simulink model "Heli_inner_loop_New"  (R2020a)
settings: Solver=FixedStepDiscrete  StartTime=0.0  StopTime=10.0  FixedStep=0.01  RelTol=1e-3  EnableMultiTasking=on
libraries: HeliLibrary_New x3, simulink x1

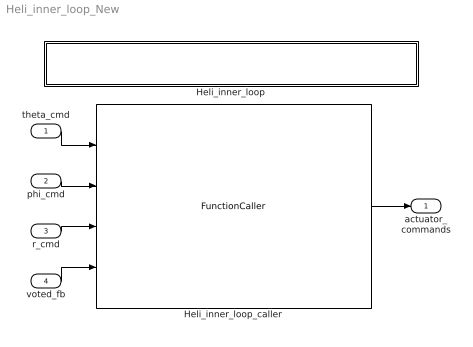
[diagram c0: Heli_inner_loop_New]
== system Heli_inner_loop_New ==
  theta_cmd : Inport  OutMin=-30  OutMax=30  OutDataTypeStr=double  PortDimensions=1  SampleTime=0.01
  phi_cmd : Inport  Port=2  OutMin=-30  OutMax=30  OutDataTypeStr=double  PortDimensions=1  SampleTime=0.01
  r_cmd : Inport  Port=3  OutMin=-30  OutMax=30  OutDataTypeStr=double  PortDimensions=1  SampleTime=0.01
  voted_fb : Inport  Port=4  OutMin=-180  OutMax=180  OutDataTypeStr=double  PortDimensions=5  SampleTime=0.01
  Heli_inner_loop : Subsystem  TreatAsAtomicUnit=on
  Heli_inner_loop_caller : FunctionCaller  FunctionPrototype=actuator_commands = Heli_inner_loop(theta_cmd,phi_cmd,r_cmd,voted_fb)
  actuator_commands : Outport  VectorParamsAs1DForOutWhenUnconnected=off
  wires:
  voted_fb/1 -> Heli_inner_loop_caller/4
  r_cmd/1 -> Heli_inner_loop_caller/3
  phi_cmd/1 -> Heli_inner_loop_caller/2
  theta_cmd/1 -> Heli_inner_loop_caller/1
  Heli_inner_loop_caller/1 -> actuator_commands/1

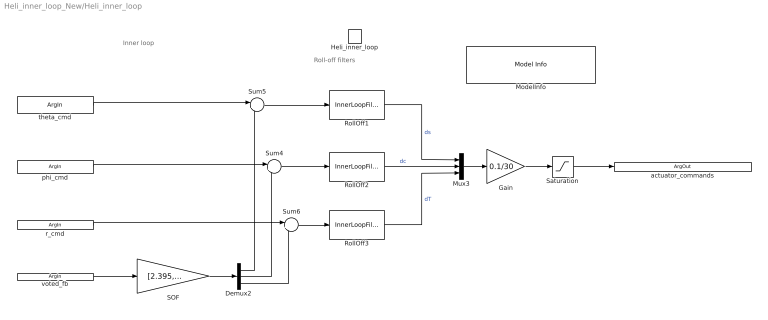
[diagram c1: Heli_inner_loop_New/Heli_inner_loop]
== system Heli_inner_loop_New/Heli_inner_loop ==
  note: Roll-off filters
  note: Inner loop
  Heli_inner_loop : TriggerPort  TriggerType=function-call  IsSimulinkFunction=on  FunctionName=Heli_inner_loop  FunctionVisibility=scoped  VariantControl=Variant  PortDimensions=1
  Demux2 : Demux  Outputs=3
  Gain : Gain  Gain=0.1/30
  ModelInfo : simulink/Model-Wide Utilities/Model Info  Frame=on  DisplayStringWithTags=|  HorizontalTextAlignment=Center  LeftAlignmentValue=0.5
      | Model Name: %<ModelName>
      | Model Version: %<ModelVersion>
      | Last Modified: %<LastModificationDate>
      | 
      | Copyright 2016 The MathWorks, Inc.
  Mux3 : Mux  Inputs=3
  RollOff1 : HeliLibrary_New/InnerLoopFilter  Tag=FilterWizardSubSystem  SystemSampleTime=-1  Latency=0  AutoFrameSizeCalculation=off
  RollOff2 : HeliLibrary_New/InnerLoopFilter  Tag=FilterWizardSubSystem  SystemSampleTime=-1  Latency=0  AutoFrameSizeCalculation=off
  RollOff3 : HeliLibrary_New/InnerLoopFilter  Tag=FilterWizardSubSystem  SystemSampleTime=-1  Latency=0  AutoFrameSizeCalculation=off
  SOF : Gain  Gain=[2.395, -0.3609, -0.002145, 0.8087, -0.0205; -0.1427, -1.115, 0.04573, -0.04318, -0.1007; -0.02792, -0.02229, -2.025, -0.06152, 0.03151;]  Multiplication=Matrix(K*u) (u vector)
  Saturation : Saturate  UpperLimit=0.1  LowerLimit=-0.1
  Sum4 : Sum  Inputs=|+-
  Sum5 : Sum  Inputs=|+-
  Sum6 : Sum  Inputs=|+-
  theta_cmd : ArgIn  OutMin=-30  OutMax=30  ArgumentName=theta_cmd
  phi_cmd : ArgIn  Port=2  OutMin=-30  OutMax=30  ArgumentName=phi_cmd
  r_cmd : ArgIn  Port=3  OutMin=-30  OutMax=30  ArgumentName=r_cmd
  voted_fb : ArgIn  Port=4  OutMin=-180  OutMax=180  PortDimensions=5  ArgumentName=voted_fb
  actuator_commands : ArgOut  PortDimensions=3  ArgumentName=actuator_commands
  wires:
  Demux2/3 -> Sum6/2
  voted_fb/1 -> SOF/1
  Saturation/1 -> actuator_commands/1
  r_cmd/1 -> Sum6/1
  Demux2/1 -> Sum5/2
  Demux2/2 -> Sum4/2
  RollOff1/1 -> Mux3/1  "ds"
  RollOff3/1 -> Mux3/3  "dT"
  theta_cmd/1 -> Sum5/1
  Gain/1 -> Saturation/1
  Sum5/1 -> RollOff1/1
  RollOff2/1 -> Mux3/2  "dc"
  SOF/1 -> Demux2/1
  Mux3/1 -> Gain/1
  Sum6/1 -> RollOff3/1
  Sum4/1 -> RollOff2/1
  phi_cmd/1 -> Sum4/1
